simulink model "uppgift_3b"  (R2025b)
settings: Solver=VariableStepAuto  StartTime=0.0  StopTime=10.0  RelTol=1e-3
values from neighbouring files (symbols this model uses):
  m_dot_end = 14*1e-3    (= 0.014)    [Lektion_2.m]
  m_dot_start = 12*1e-3    (= 0.012)    [Lektion_2.m]
  R = 280    [Lektion_2.m]
  T_i = 320    [Lektion_2.m]
  tau_th = 1/0.1    (= 10)    [Lektion_2.m]
  V_i = 2/1e3    (= 0.002)    [Lektion_2.m]
undefined symbols (not defined in the file or in its folder): p_im

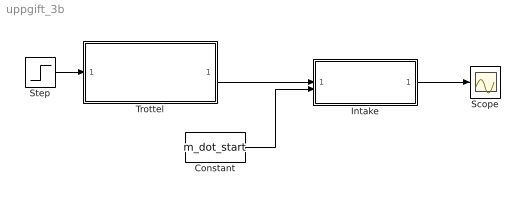
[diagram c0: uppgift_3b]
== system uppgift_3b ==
  Constant : Constant  Value=m_dot_start
  Intake : Subsystem
  Scope : Scope
  Step : Step  Time=3  Before=m_dot_start  After=m_dot_end  SampleTime=0
  Trottel : Subsystem
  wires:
  Trottel/1(m_at [kg/s]) -> Intake/1(m_at [kg/s])
  Constant/1 -> Intake/2(m_ac [kg/s])
  Intake/1(p_im [Pa]) -> Scope/1
  Step/1 -> Trottel/1(m_at,raf [kg/s])

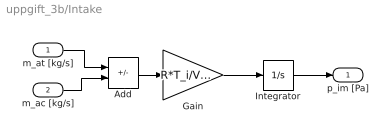
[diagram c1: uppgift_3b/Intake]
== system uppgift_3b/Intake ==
  m_at [kg/s] : Inport
  m_ac [kg/s] : Inport  Port=2
  Add : Sum  Inputs=+-
  Gain : Gain  Gain=R*T_i/V_i
  Integrator : Integrator  InitialCondition=p_im
  p_im [Pa] : Outport
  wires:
  Integrator/1 -> p_im [Pa]/1
  Gain/1 -> Integrator/1
  m_ac [kg/s]/1 -> Add/2
  m_at [kg/s]/1 -> Add/1
  Add/1 -> Gain/1

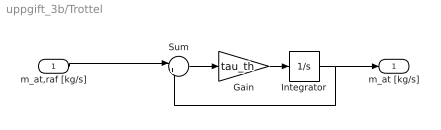
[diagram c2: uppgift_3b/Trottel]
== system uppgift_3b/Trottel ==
  m_at,raf [kg/s] : Inport
  Gain : Gain  Gain=tau_th
  Integrator : Integrator  InitialCondition=m_dot_start
  Sum : Sum  Inputs=|+-
  m_at [kg/s] : Outport
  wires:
  Sum/1 -> Gain/1
  Integrator/1 -> m_at [kg/s]/1, Sum/2
  m_at,raf [kg/s]/1 -> Sum/1
  Gain/1 -> Integrator/1
